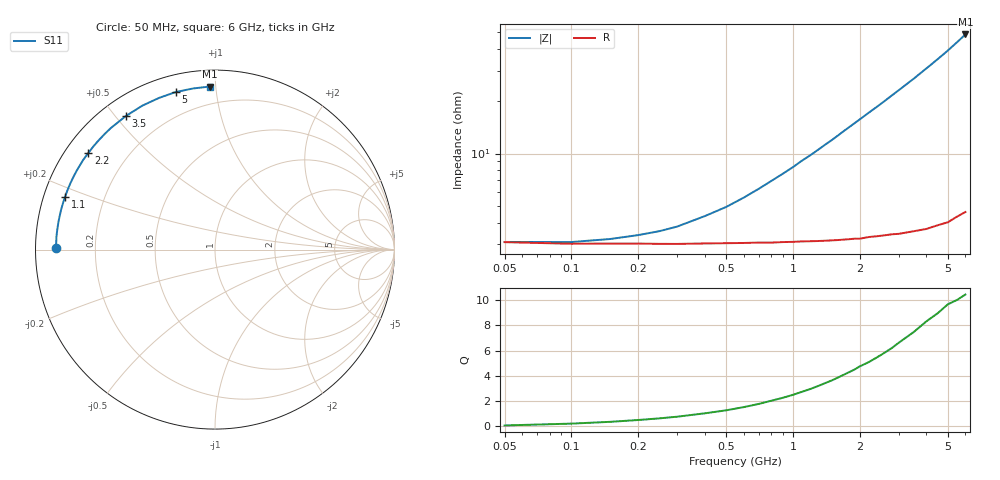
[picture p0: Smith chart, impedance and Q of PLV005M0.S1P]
! Infineon Technologies  Discrete & RF Semiconductors
! BAR 64-04W /-05W /-06W
! Si PIN Diode in SOT323
! IF = 5 mA
! S-Parameters:  October  2008
# GHz  S  MA  R  50
!  f  S11
! GHz  MAG  ANG
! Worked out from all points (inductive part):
!   34 points, 50 MHz to 6 GHz, reference 50 ohm
!   read as one part to ground: L = 1.23 nH near 1.3 GHz
!   highest Q = 10.4 at 6 GHz (marker M1), where L = 1.28 nH
!   S11 on the Smith chart (normalised r, x): 50 MHz: 0.06, +0.00; 1.1 GHz: 0.06, +0.17; 2.2 GHz: 0.07, +0.34; 3.5 GHz: 0.07, +0.53; 5 GHz: 0.08, +0.78; 6 GHz: 0.09, +0.96
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0.05  0.8834 179.5
0.1  0.8858 178.5
0.2  0.8856 176.5
0.3  0.8862 174.7
0.4  0.8858 172.8
0.5  0.8856 171.1
0.6  0.8856 169.3
0.8  0.8858 165.7
1  0.8856 162.3
1.1  0.8855 160.5
1.2  0.8858 158.9
1.3  0.8861 157.2
1.4  0.8864 155.5
1.5  0.8865 153.9
1.6  0.8868 152.2
1.7  0.887 150.5
2  0.8883 145.7
2.2  0.8878 142.6
2.4  0.8886 139.6
2.6  0.8894 136.6
2.8  0.8902 133.6
3  0.892 130.7
3.5  0.8946 123.7
4  0.8984 116.8
4.5  0.9008 110.3
5  0.9046 104.0
5.5  0.906 97.8
6  0.9088 91.9
